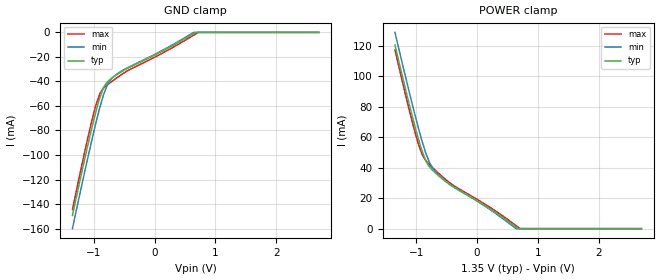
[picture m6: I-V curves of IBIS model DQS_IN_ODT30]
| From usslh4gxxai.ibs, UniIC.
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| MODEL DQS_IN_ODT30 (Data Strobe Input with 30ohm ODT, 800-2133Mbps)
[Model]   DQS_IN_ODT30
Model_type   Input
Vinl = 545.000mV
Vinh = 805.000mV
|   typ   min   max
|C_comp   1.105pF   1.047pF   1.139pF
C_comp_power_clamp   0.5525pF   0.5235pF   0.5695pF
C_comp_gnd_clamp   0.5525pF   0.5235pF   0.5695pF
| Note: C_comp changes when the ODT circuit is enabled.
[Model Spec]
| Input threshold voltage corners
Vinl   0.5450V   0.5115V   0.5825V
Vinh   0.8050V   0.7715V   0.8425V
| Dynamic Overshoot Parameters from DDR3L Specification
|D_overshoot_ampl_h   0.40   NA   NA
|D_overshoot_ampl_l   0.40   NA   NA
|D_overshoot_area_h   0.11n   NA   NA
|D_overshoot_area_l   0.11n   NA   NA
[Receiver Thresholds]
|Vth   =  0.675V
|Vth_min  =  0.6615V
|Vth_max  =  0.6885V
|Vinh_ac  =  0.130V
|Vinh_dc  =  0.090V
|Vinl_ac  = -0.130V
|Vinl_dc  = -0.090V
|Tslew_ac =  5.000ns |Not specified, so set to high value
|Threshold_sensitivity = 0.50
|Reference_supply Power_clamp_ref
|NOTE: If using the IBISCHK 4.2.1 or older parser, Differential receiver
|threshold parameters must be commented out because the parser generates
|errors for multiple differential models.
Vcross_low   = 0.545V
Vcross_high  = 0.805V
Vdiff_ac   = 260mV
Vdiff_dc   = 180mV
Tdiffslew_ac = 10.000ns |Not specified, so set to high value
[Voltage Range]   1.3500V   1.2830V   1.4250V
[POWER Clamp Reference]   1.3500V   1.2830V   1.4250V
[Temperature Range]   45.0   95.0   -40.0
[GND Clamp]
|   Voltage   I(typ)   I(min)   I(max)
-1.35V    -149.3mA   -160.1mA   -144.5mA
-1.085V   -89.13mA   -99.43mA   -83.24mA
-960mV    -63.79mA   -72.88mA   -58.43mA
-900mV    -53.32mA   -61.2mA    -49.97mA
-840mV    -45.07mA   -50.91mA   -45.48mA
-775mV    -40.35mA   -42.64mA   -42.69mA
-655mV    -35.63mA   -35.25mA   -38.25mA
-425mV    -28.77mA   -28.28mA   -30.77mA
65mV      -16.87mA   -16.28mA   -18.57mA
640mV     -1.008mA   -45.78uA   -2.34mA
720mV     0A         0A         0A
2.7V      0A         0A         0A
[POWER Clamp]
|   Voltage   I(typ)   I(min)   I(max)
-1.35V    120.3mA    128.6mA    117.2mA
-1.085V   76.62mA    84.61mA    72.84mA
-965mV    58.82mA    65.95mA    55.43mA
-900mV    50.41mA    56.66mA    48.33mA
-845mV    44.56mA    49.63mA    44.71mA
-775mV    40.18mA    42.71mA    41.67mA
-655mV    35.46mA    36.07mA    37.1mA
-525mV    31.14mA    31.44mA    32.5mA
200mV     13.25mA    12.84mA    14.25mA
640mV     1.022mA    41.43uA    1.966mA
705mV     0A         0A         0A
2.7V      0A         0A         0A
